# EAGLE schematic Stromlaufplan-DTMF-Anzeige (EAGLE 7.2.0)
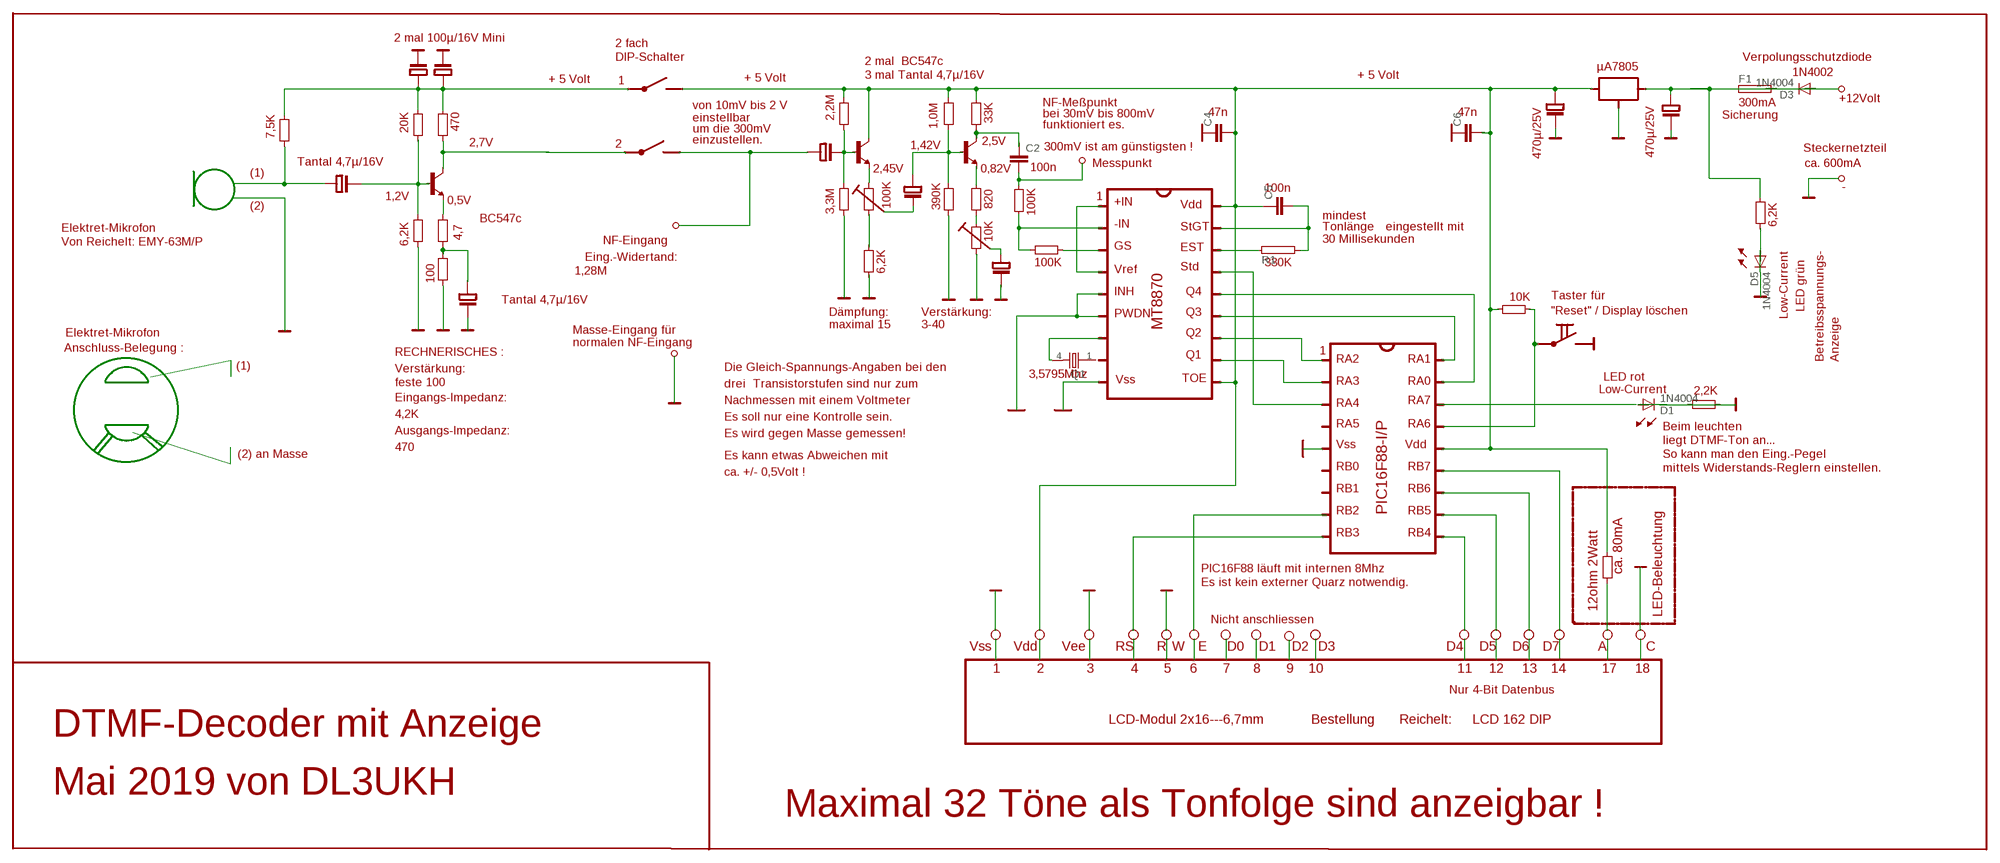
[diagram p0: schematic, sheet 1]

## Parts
C2  C2,5-3  [C2.5-3]
C4  C2,5-3  [C2.5-3]
C5  C2,5-3  [C2.5-3]
C6  C2,5-3  [C2.5-3]
D1  1N4004  [DO41-10]
D3  1N4004  [DO41-10]
D5  1N4004  [DO41-10]
F1  19559  [19559]
Q1  86SMX  [86SMX]
R1  RHS10  [HS10]

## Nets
N$6: Q1.4
N$12: R1.1
N$13: C5.2 R1.2
N$14: C2.2
N$19: C5.1
N$25: D1.A D1.C
N$34: D5.A D5.C
N$35: D3.C
N$46: C4.2 C6.2
N$47: D3.A F1.1 F1.2
N$58: C2.1
Unconnected: C4.1 C6.1 Q1.1

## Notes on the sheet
- 2 mal 100µ/16V Mini
- 2 fach
- DIP-Schalter | Verpolungsschutzdiode
- 2 mal  BC547c
- + 5 Volt | + 5 Volt | µA7805
- + 5 Volt | 1N4002
- 3 mal Tantal 4,7µ/16V
- 1
- +12Volt
- von 10mV bis 2 V | NF-Meßpunkt | 300mA
- bei 30mV bis 800mV | 47n | 47n | Sicherung
- einstellbar | 2,2M | 33K
- 470 | 1,0M | funktioniert es.
- 20K | um die 300mV
- 7,5K
- 2,7V | einzustellen. | 2,5V
- 2 | 1,42V | 300mV ist am günstigsten !
- Steckernetzteil
- 470µ/25V | 470µ/25V
- Tantal 4,7µ/16V | Messpunkt | ca. 600mA
- 2,45V | 0,82V | 100n
- (1)
- 100n | -
- 1,2V | 1
- 0,5V | +IN
- (2) | 100K | 390K | 820 | Vdd
- BC547c | 3,3M | 100K
- mindest
- -IN | 6,2K
- Elektret-Mikrofon | StGT | Tonlänge | eingestellt mit
- 4,7 | 10K | 30 Millisekunden
- Von Reichelt: EMY-63M/P | 6,2K | NF-Eingang
- Eing.-Widertand: | GS | EST
- LED grün
- 1,28M | 100K | 330K
- 6,2K | Vref | Std
- 100
- Tantal 4,7µ/16V | INH | Q4 | 10K
- Taster für
- Dämpfung: | Verstärkung: | PWDN | Q3 | "Reset" / Display löschen
- Low-Current
- maximal 15 | 3-40 | MT8870
- Elektret-Mikrofon | Masse-Eingang für | Q2
- normalen NF-Eingang
- Anschluss-Belegung : | 1
- RECHNERISCHES : | Q1
- RA2 | RA1 | Betreibsspannungs- | Anzeige
- (1) | Verstärkung: | Die Gleich-Spannungs-Angaben bei den
- 3,5795Mhz | LED rot
- Vss | TOE | RA3 | RA0 | Low-Current
- feste 100 | drei  Transistorstufen sind nur zum | 2,2K
- Eingangs-Impedanz: | Nachmessen mit einem Voltmeter | RA7
- RA4
- 4,2K | Es soll nur eine Kontrolle sein.
- RA5 | RA6 | Beim leuchten
- Ausgangs-Impedanz: | Es wird gegen Masse gemessen!
- liegt DTMF-Ton an...
- 470 | Vss | Vdd
- (2) an Masse | Es kann etwas Abweichen mit | So kann man den Eing.-Pegel
- RB0 | RB7 | mittels Widerstands-Reglern einstellen.
- ca. +/- 0,5Volt !
- RB1 | RB6
- RB2 | PIC16F88-I/P | RB5
- RB3 | RB4
- PIC16F88 läuft mit internen 8Mhz | ca. 80mA
- Es ist kein externer Quarz notwendig.
- 12ohm 2Watt
- LED-Beleuchtung
- Nicht anschliessen
- Vss | Vdd | Vee | RS | R | W | E | D0 | D1 | D2 | D3 | D4 | D5 | D6 | D7 | A | C
- 1 | 2 | 3 | 4 | 5 | 6 | 7 | 8 | 9 | 10 | 11 | 12 | 13 | 14 | 17 | 18
- Nur 4-Bit Datenbus
- LCD-Modul 2x16---6,7mm | Bestellung | Reichelt: | LCD 162 DIP
- DTMF-Decoder mit Anzeige
- Mai 2019 von DL3UKH
- Maximal 32 Töne als Tonfolge sind anzeigbar !

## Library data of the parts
C2 C4-C6 = capacitor-wima:C: CAPACITOR
D1 D3 D5 = diode:1N4004: DIODE
F1 = fuse:19559: FUSE HOLDER
Q1 = crystal:86SMX: CRYSTAL
R1 = resistor-power:R: Power Resitor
